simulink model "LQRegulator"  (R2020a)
settings: Solver=VariableStepAuto  StartTime=0.0  StopTime=10.0  RelTol=1e-3
InitFcn:
  | initParams
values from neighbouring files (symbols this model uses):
  A = [-1 -2 1;0 -9 -1;0 0 -1]    [initParams.m]
  B = [0 1;0 0; 1 0]    [initParams.m]
  C = [0 0 1]    [initParams.m]
  ud = [9;0]    [initParams.m]
  x0 = [10;-10]    [initParams.m]
  xd = [11;-1;9]    [initParams.m]
undefined symbols (not defined in the file or in its folder): K

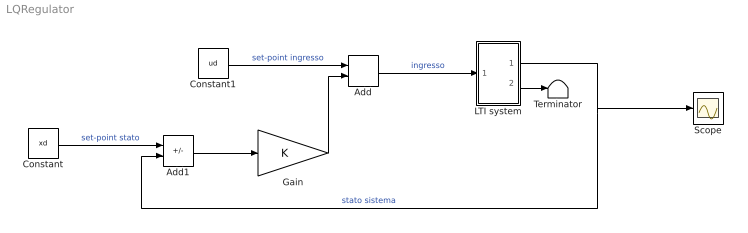
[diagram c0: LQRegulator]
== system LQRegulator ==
  Add : Sum
  Add1 : Sum  Inputs=+-
  Constant : Constant  Value=xd
  Constant1 : Constant  Value=ud
  Gain : Gain  Gain=K  Multiplication=Matrix(K*u) (u vector)
  LTI system : Subsystem
  Scope : Scope
  Terminator : Terminator
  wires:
  Constant1/1 -> Add/1  "set-point ingresso"
  Add/1 -> LTI system/1(u)  "ingresso"
  LTI system/2(y) -> Terminator/1
  Constant/1 -> Add1/1  "set-point stato"
  Add1/1 -> Gain/1
  Gain/1 -> Add/2
  LTI system/1(x) -> Add1/2, Scope/1  "stato sistema"

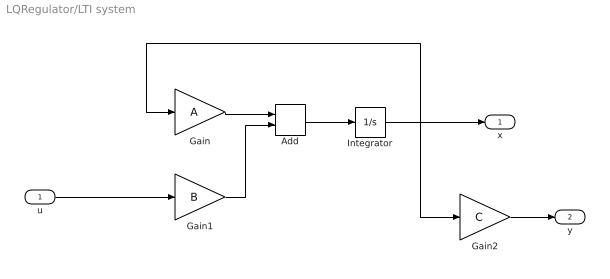
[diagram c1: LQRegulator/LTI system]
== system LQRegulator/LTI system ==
  u : Inport
  Add : Sum
  Gain : Gain  Gain=A  Multiplication=Matrix(K*u) (u vector)
  Gain1 : Gain  Gain=B  Multiplication=Matrix(K*u) (u vector)
  Gain2 : Gain  Gain=C  Multiplication=Matrix(K*u) (u vector)
  Integrator : Integrator  InitialCondition=x0
  x : Outport
  y : Outport  Port=2
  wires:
  Gain2/1 -> y/1
  Gain1/1 -> Add/2
  Integrator/1 -> x/1, Gain2/1, Gain/1
  Gain/1 -> Add/1
  Add/1 -> Integrator/1
  u/1 -> Gain1/1
